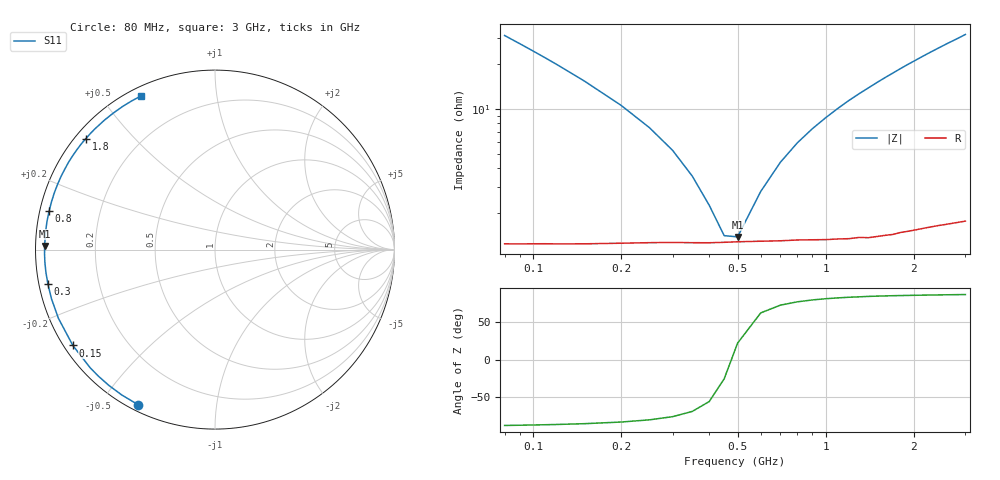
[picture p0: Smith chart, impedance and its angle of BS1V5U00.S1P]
! SIEMENS Small Signal Semiconductors
! BB640
! Si Tuning Diode in SOD323
! VR = 1.5 V
! S-Parameters:  July  1993
# GHz  S  MA  R  50
!  f  S11
! GHz  MAG  ANG
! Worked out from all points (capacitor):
!   33 points, 80 MHz to 3 GHz, reference 50 ohm
!   read as one part to ground: C = 62.5 pF near 80 MHz
!   lowest |Z| = 1.39 ohm at 500 MHz (marker M1)
!   series resonance near 476.9 MHz, so ESL is about 1.8 nH
!   S11 on the Smith chart (normalised r, x): 80 MHz: 0.03, -0.62; 150 MHz: 0.03, -0.31; 300 MHz: 0.03, -0.10; 800 MHz: 0.03, +0.12; 1.8 GHz: 0.03, +0.37; 3 GHz: 0.04, +0.63
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0.08  0.9644 -116.5
0.09  0.9622 -122.7
0.1  0.9603 -128.0
0.11  0.9588 -132.6
0.12  0.9577 -136.6
0.15  0.9552 -146.0
0.2  0.9527 -156.3
0.25  0.9513 -163.2
0.3  0.9506 -168.3
0.35  0.9505 -172.4
0.4  0.9504 -175.7
0.45  0.95 -178.6
0.5  0.9496 178.8
0.6  0.9493 174.3
0.7  0.9492 170.4
0.8  0.9489 166.8
0.9  0.9491 163.5
1  0.9494 160.4
1.2  0.9497 154.5
1.4  0.9501 149.2
1.6  0.9496 144.1
1.8  0.9489 139.3
2  0.9487 134.8
2.2  0.9485 130.5
2.4  0.9486 126.5
2.6  0.9491 122.7
2.8  0.9496 119.2
3  0.9503 115.7
